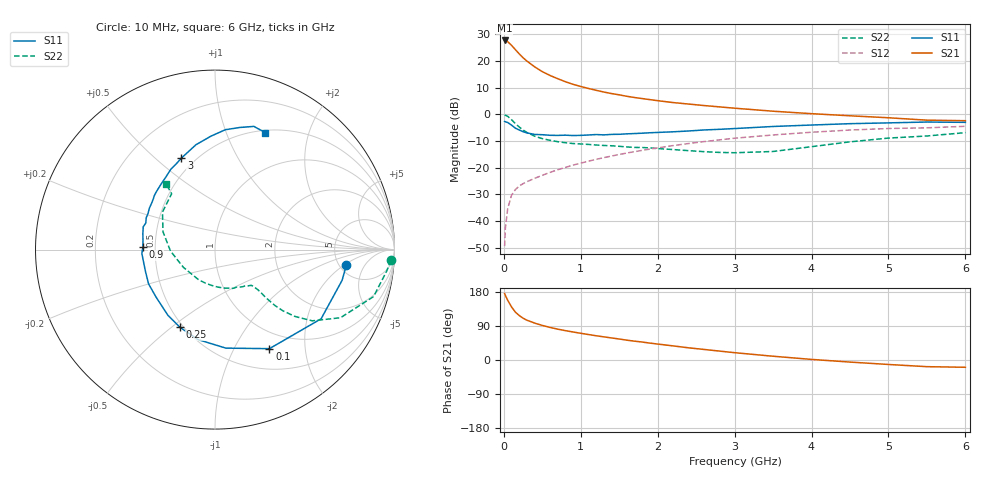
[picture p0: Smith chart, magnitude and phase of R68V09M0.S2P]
! SIEMENS Small Signal Semiconductors
! BFR193
! Si NPN RF Bipolar Junction Transistor in SOT23
! VCE = 8 V  IC = 9 mA
! Common Emitter S-Parameters:  May  1996
# GHz  S  MA  R  50
!  f  S11  S21  S12  S22
! GHz  MAG  ANG  MAG  ANG  MAG  ANG  MAG  ANG
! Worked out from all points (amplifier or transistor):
!   36 points, 10 MHz to 6 GHz, reference 50 ohm
!   highest |S21| = 27.7 dB at 10 MHz (marker M1)
!   |S21| within 3 dB of that: start of sweep to 136.4 MHz
!   unconditionally stable (mu >= 1): 793.7 MHz to 2.04 GHz
!   at 250 MHz: K = 0.60, MSG = 23.6 dB, |S12| = -26.0 dB
!   at 1.4 GHz: K = 1.04, MAG = 10.5 dB, |S12| = -15.6 dB
!   at 6 GHz: K = 0.94, MSG = 1.0 dB, |S12| = -4.5 dB
!   S11 on the Smith chart (normalised r, x): 10 MHz: 5.72, -2.21; 100 MHz: 0.76, -1.40; 250 MHz: 0.48, -0.54; 900 MHz: 0.43, +0.01; 3 GHz: 0.42, +0.61; 6 GHz: 0.53, +1.38
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0.01  0.7367 -6.9  24.28 175.3  0.0034 85.1  0.9814 -3.4
0.02  0.7285 -13.6  24.26 170.4  0.0074 85.1  0.9653 -6.9
0.05  0.7058 -33.1  23.05 157.7  0.0171 75.3  0.9216 -16.5
0.1  0.6298 -61.2  19.69 140.1  0.0306 65.3  0.7955 -28.5
0.15  0.5523 -83.7  16.34 126.3  0.0391 58.3  0.6719 -36.2
0.2  0.5102 -100.7  13.63 117.4  0.0455 55.7  0.5805 -39.9
0.25  0.4748 -114.3  11.52 110.3  0.0504 54.4  0.5105 -42.0
0.3  0.4502 -125.7  9.973 105.0  0.0549 54.9  0.4585 -43.0
0.4  0.4217 -141.1  7.789 97.4  0.0634 56.2  0.391 -43.4
0.5  0.4165 -152.7  6.316 91.2  0.0723 57.6  0.3514 -43.1
0.6  0.4061 -162.4  5.368 86.0  0.082 59.0  0.3273 -43.1
0.7  0.404 -170.4  4.663 81.4  0.0918 60.2  0.3087 -43.5
0.9  0.4018 178.1  3.658 73.9  0.1122 61.6  0.2845 -44.5
1.1  0.4115 167.6  3.061 67.2  0.133 61.9  0.2738 -47.6
1.3  0.413 159.0  2.623 61.1  0.155 61.7  0.2618 -50.8
1.6  0.4322 147.8  2.183 52.3  0.1891 60.1  0.2458 -58.2
2.2  0.4721 129.7  1.666 37.2  0.2605 55.0  0.2196 -77.3
3  0.5432 110.1  1.307 19.3  0.3579 44.9  0.1913 -118.2
3.5  0.5938 100.3  1.147 9.9  0.4119 37.6  0.2019 -150.6
4.5  0.6703 85.1  0.942 -5.5  0.5096 22.7  0.3062 161.1
5.5  0.7198 72.5  0.78 -17.6  0.5603 7.1  0.3941 127.8
6  0.7097 66.8  0.762 -19.2  0.5986 2.6  0.4551 126.7
